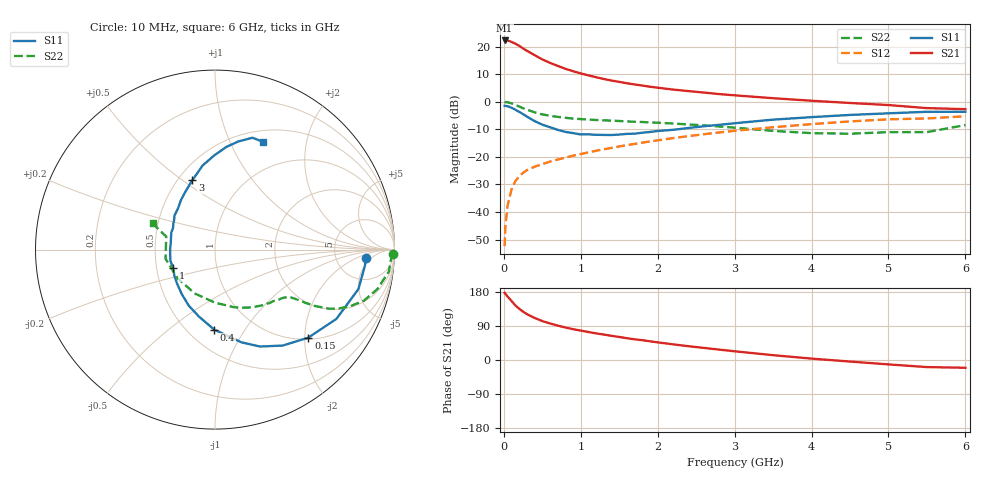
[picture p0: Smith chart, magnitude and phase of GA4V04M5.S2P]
! Infineon Technologies  Discrete & RF Semiconductors
! BF775
! Si NPN RF Bipolar Junction Transistor in SOT23
! VCE = 4 V  IC = 4.5 mA
! Common Emitter S-Parameters:  May  1996
# GHz  S  MA  R  50
!  f  S11  S21  S12  S22
! GHz  MAG  ANG  MAG  ANG  MAG  ANG  MAG  ANG
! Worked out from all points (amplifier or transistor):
!   36 points, 10 MHz to 6 GHz, reference 50 ohm
!   highest |S21| = 22.2 dB at 10 MHz (marker M1)
!   |S21| within 3 dB of that: start of sweep to 256.2 MHz
!   unconditionally stable (mu >= 1): 847.1 MHz to 3.346 GHz
!   at 250 MHz: K = 0.45, MSG = 22.6 dB, |S12| = -25.8 dB
!   at 1.4 GHz: K = 1.12, MAG = 10.1 dB, |S12| = -16.8 dB
!   at 6 GHz: K = 0.95, MSG = 1.3 dB, |S12| = -5.3 dB
!   S11 on the Smith chart (normalised r, x): 10 MHz: 11, -3; 150 MHz: 1.04, -2.08; 400 MHz: 0.66, -0.74; 1 GHz: 0.61, -0.13; 3 GHz: 0.59, +0.55; 6 GHz: 0.63, +1.33
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0.01  0.8432 -3.1  12.92 177.4  0.0024 91.3  0.9938 -1.3
0.02  0.8399 -6.2  12.91 174.6  0.0055 84.8  0.9828 -2.9
0.05  0.8288 -15.4  12.91 167.2  0.0134 83.1  0.976 -7.2
0.1  0.7789 -29.7  12.15 155.7  0.0257 74.8  0.9318 -13.6
0.15  0.715 -43.3  11.29 144.0  0.0364 68.1  0.8773 -18.9
0.2  0.6543 -54.8  10.32 135.2  0.0445 64.0  0.8171 -22.7
0.25  0.5955 -65.1  9.258 127.6  0.0513 60.4  0.7641 -25.4
0.3  0.5371 -74.1  8.392 121.0  0.0573 58.4  0.7187 -27.3
0.4  0.4455 -90.6  7 111.1  0.0663 56.0  0.6409 -29.4
0.5  0.3836 -103.5  5.855 102.7  0.0739 55.3  0.5891 -30.4
0.6  0.3448 -115.1  5.07 96.5  0.0821 54.5  0.5569 -30.9
0.7  0.3092 -126.8  4.466 90.8  0.0893 55.3  0.531 -31.4
0.8  0.2838 -138.2  3.96 85.8  0.097 55.6  0.5113 -31.9
1  0.255 -156.6  3.26 77.6  0.1124 56.5  0.4845 -32.9
1.1  0.2558 -165.9  3.001 73.8  0.1208 56.7  0.4749 -34.1
1.6  0.261 159.0  2.162 57.5  0.1634 56.1  0.4397 -40.3
2.2  0.3093 131.6  1.66 41.3  0.2189 53.3  0.4023 -51.0
3  0.4071 108.0  1.307 23.0  0.2969 46.2  0.3389 -71.5
3.5  0.4734 98.4  1.158 12.7  0.3443 40.6  0.2956 -90.1
4.5  0.5762 83.6  0.949 -4.1  0.4396 28.0  0.263 -142.8
5.5  0.6572 71.5  0.766 -18.7  0.4974 12.9  0.281 165.1
6  0.6576 66.2  0.733 -20.5  0.5444 8.7  0.3772 157.3
